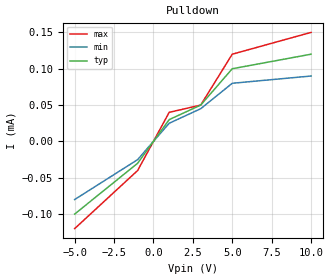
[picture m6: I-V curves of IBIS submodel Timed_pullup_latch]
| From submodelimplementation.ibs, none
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| ********* Off delay test. example taken from Bird 57 ****
| Complete Pullup Timed Latch Example:
[Submodel]   Timed_pullup_latch
Submodel_type   Bus_hold
[Submodel Spec]
|   Subparameter   typ   min   max
V_trigger_r   3.1   2.6   4.6  | Rising edge trigger
   | Values could be set out
   | of range to disable the
   | trigger
V_trigger_f   1.3   1.2   1.4  | Falling edge trigger
Off_delay   3n   5n   2n   | Delay to turn off the
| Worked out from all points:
|   slope of the pulldown table from 0 to 0.3 V, typ, clamps not added: 33.3 kohm
   | pullup table
| Note that if the input signal goes above the V_trigger_r value, the
| pulldown structure will turn off even if the timer didn't expire yet.
|   typ   min   max
| [Voltage Range]   5.0   4.5   5.5
| Note, the actual voltage range and reference voltages are inherited from
| the top-level model.
[Pulldown]
-5V       -100uA     -80uA      -120uA
-1V       -30uA      -25uA      -40uA
0V        0A         0A         0A
1V        30uA       25uA       40uA
3V        50uA       45uA       50uA
5V        100uA      80uA       120uA
10V       120uA      90uA       150uA
| [Pullup] table is omitted to signal Open_source functionality
[Ramp]
|   typ   min   max
dV/dt_r   2.0/0.50n   2.0/0.75n   2.0/0.35n
dV/dt_f   2.0/0.50n   2.0/0.75n   2.0/0.35n
R_load = 500
